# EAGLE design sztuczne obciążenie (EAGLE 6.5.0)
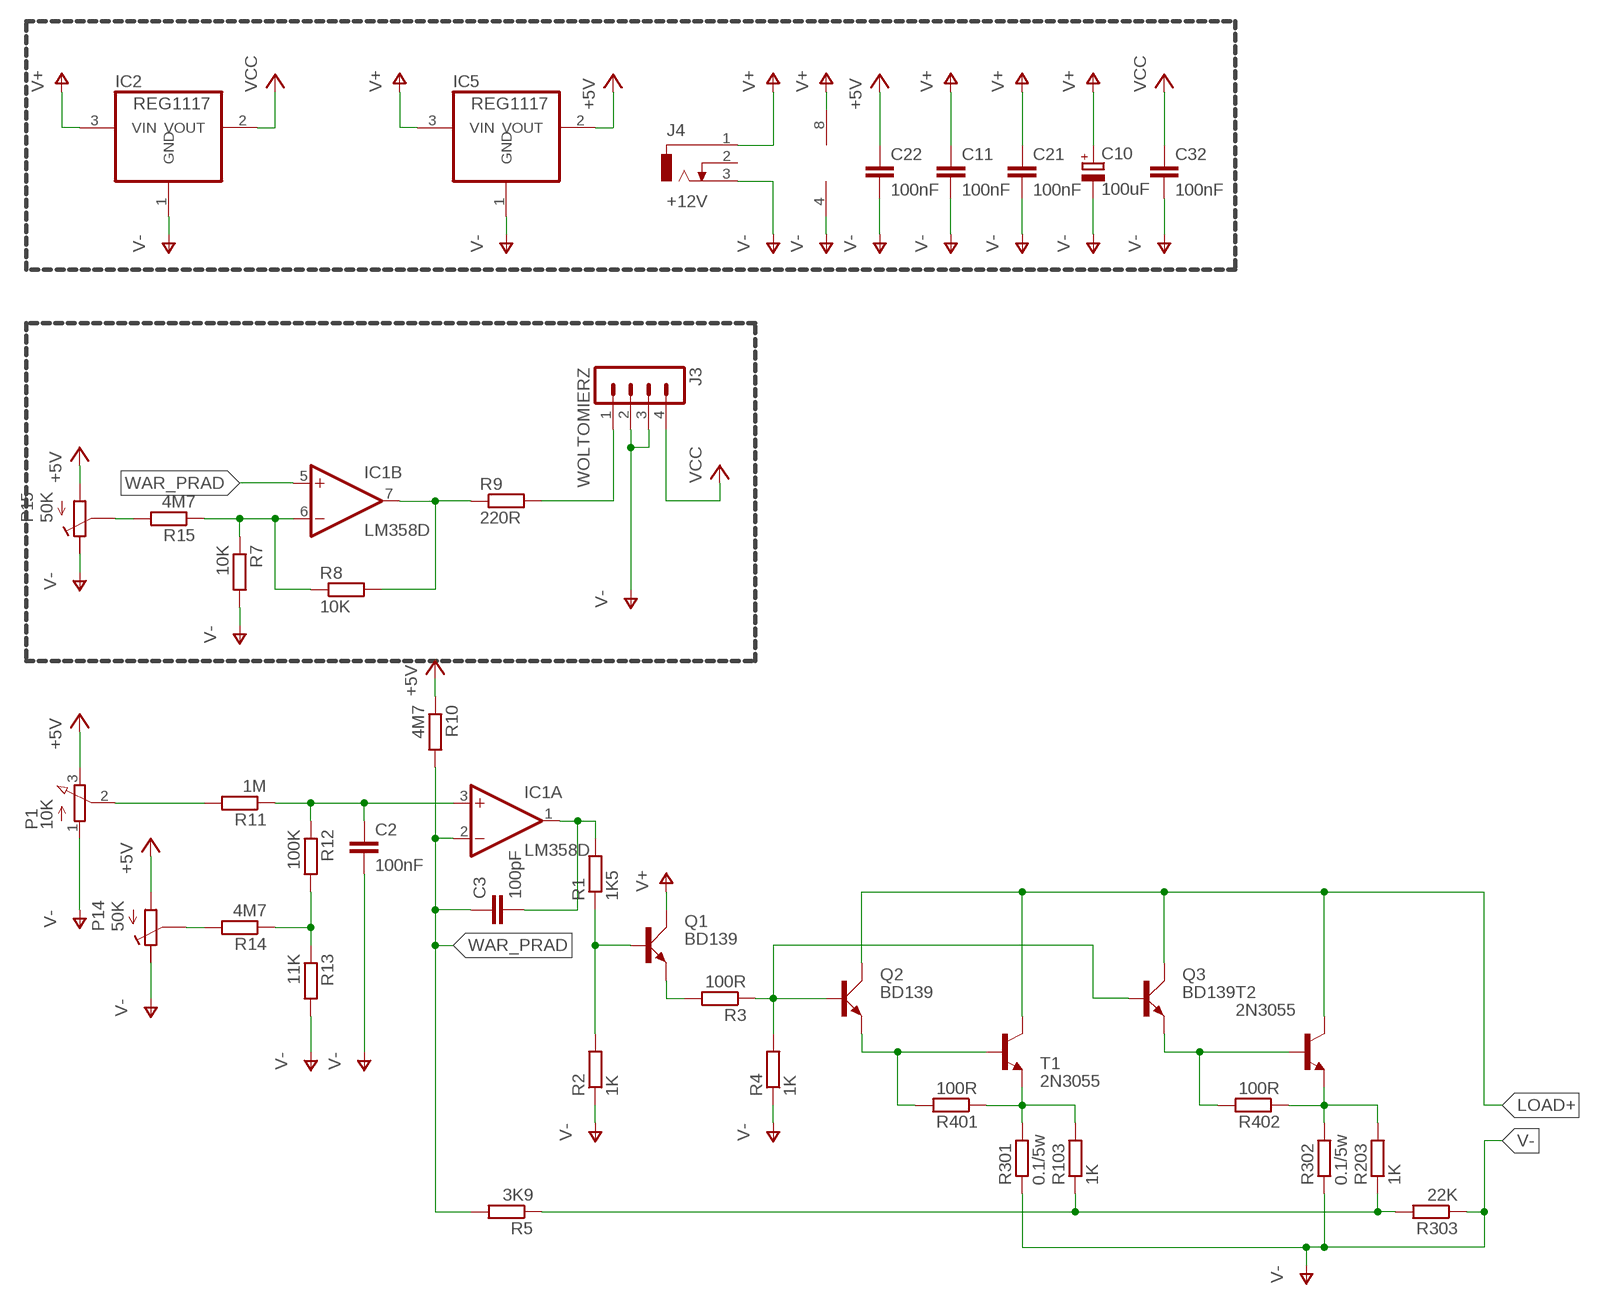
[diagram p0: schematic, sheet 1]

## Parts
C2  100nF  C-EU050-025X075  [C050-025X075]
C3  100pF  C-EUC1206K  [C1206K]
C10  100uF  CPOL-EUE5-10.5  [E5-10,5]
C11  100nF  C-EU050-025X075  [C050-025X075]
C21  100nF  C-EU050-025X075  [C050-025X075]
C22  100nF  C-EU050-025X075  [C050-025X075]
C32  100nF  C-EU050-025X075  [C050-025X075]
IC1  LM358D  [SO08]
IC2  REG1117  [SOT223]
IC5  REG1117  [SOT223]
J3  WOLTOMIERZ  MA04-1  [MA04-1]
J4  +12V  DCJ0202  [DCJ0202]
P1  10K  3RP/1610N  [3RP/1610N]
P14  50K  POTENCJOMETR_RM-065  [RM065]
P15  50K  POTENCJOMETR_RM-065  [RM065]
Q1  BD139  [TO126AV]
Q2  BD139  [TO126AV]
Q3  BD139  [TO126AV]
R1  1K5  R-EU_0207/7  [0207/7]
R2  1K  R-EU_0207/7  [0207/7]
R3  100R  R-EU_0207/7  [0207/7]
R4  1K  R-EU_0207/7  [0207/7]
R5  3K9  R-EU_0207/7  [0207/7]
R7  10K  R-EU_0207/7  [0207/7]
R8  10K  R-EU_0207/7  [0207/7]
R9  220R  R-EU_0207/7  [0207/7]
R10  4M7  R-EU_0207/7  [0207/7]
R11  1M  R-EU_0207/7  [0207/7]
R12  100K  R-EU_0207/7  [0207/7]
R13  11K  R-EU_0207/7  [0207/7]
R14  4M7  R-EU_0207/7  [0207/7]
R15  4M7  R-EU_0207/7  [0207/7]
R103  1K  R-EU_0207/7  [0207/7]
R203  1K  R-EU_0207/7  [0207/7]
R301  0.1/5w  R-EU_0922/22  [0922/22]
R302  0.1/5w  R-EU_0922/22  [0922/22]
R303  22K  R-EU_0207/7  [0207/7]
R401  100R  R-EU_0207/7  [0207/7]
R402  100R  R-EU_0207/7  [0207/7]
T1  2N3055  [TO3]
T2  2N3055  [TO3]

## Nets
+5V: C22.1 IC5.2(VOUT) P1.3(E) P14.P$3(A) P15.P$3(A) R10.1
LOAD+: Q2.C Q3.C T1.C T1.C/(C) T2.C T2.C/(C)
N$1: R103.2 R301.2 R401.1 T1.E
N$2: R203.2 R302.2 R402.1 T2.E
N$3: Q2.B Q3.B R3.1 R4.2
N$4: Q2.E R401.2 T1.B
N$5: Q1.B R1.1 R2.2
N$7: J3.1 R9.2
N$8: C3.2 IC1.1(A:OUT) R1.2
N$9: P1.2(S) R11.2
N$10: C2.1 IC1.3(A:+IN) R11.1 R12.1
N$11: R12.2 R13.1 R14.1
N$12: Q1.E R3.2
N$13: Q3.E R402.2 T2.B
N$14: R5.1 R103.1 R203.1 R303.2
N$15: P14.P$1(S) R14.2
N$16: IC1.6(B:-IN) R7.1 R8.1 R15.1
N$17: P15.P$1(S) R15.2
N$19: IC1.7(B:OUT) R8.2 R9.1
V+: C10.+ C11.1 C21.1 IC1.8(P:V+) IC2.3(VIN) IC5.3(VIN) J4.1 Q1.C
V-: C2.2 C10.- C11.2 C21.2 C22.2 C32.2 IC1.4(P:V-) IC2.1(GND) IC5.1(GND) J3.2 J3.3 J4.3 P1.1(A) P14.P$2(E) P15.P$2(E) R2.1 R4.1 R7.2 R13.2 R301.1 R302.1 R303.1
VCC: C32.1 IC2.2(VOUT) J3.4
WAR_PRAD: C3.1 IC1.2(A:-IN) IC1.5(B:+IN) R5.2 R10.2
Unconnected: J4.2

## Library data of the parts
C2 C3 C11 C21 C22 C32 = rcl:C-EU: CAPACITOR, European symbol
C10 = rcl:CPOL-EU: POLARIZED CAPACITOR, European symbol
IC1 = linear:LM358: OP AMP also LM158; LM258; LM2904 Source: http://cache.national.com/ds/LM/LM158.pdf
IC2 IC5 = burr-brown:REG1117: 800mA and 1A Low Dropout (LDO) Positive Regulator 1.8V, 2.5V, 2.85V, 3.3V, 5V, and Adj; MPN: REG1117; OC_FARNELL: 1097566; OC_NEWARK: 14P6981
J3 = con-lstb:MA04-1: PIN HEADER; OC_FARNELL: unknown; OC_NEWARK: unknown
J4 = con-jack:DCJ0202: DC POWER JACK Source: DCJ0202.pdf; OC_FARNELL: unknown; OC_NEWARK: unknown
P1 = pot:3RP/1610N: 16mm Potentiometer one level Source: http://www.alphapotentiometers.net/html/16mm_pot_2.html
P14 P15 = POT_RM065:POTENCJOMETR_RM-065
Q1-Q3 = transistor-power:BD139: NPN TRANSISTOR
R1-R5 R7-R15 R103 R203 R301-R303 R401 R402 = resistor:R-EU_: RESISTOR, European symbol
T1 T2 = transistor:2N3055: NPN TRANSISTOR

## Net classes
1 pradowa: width 1.524 mm, clearance 0.508 mm
2 srednia: width 0.635 mm

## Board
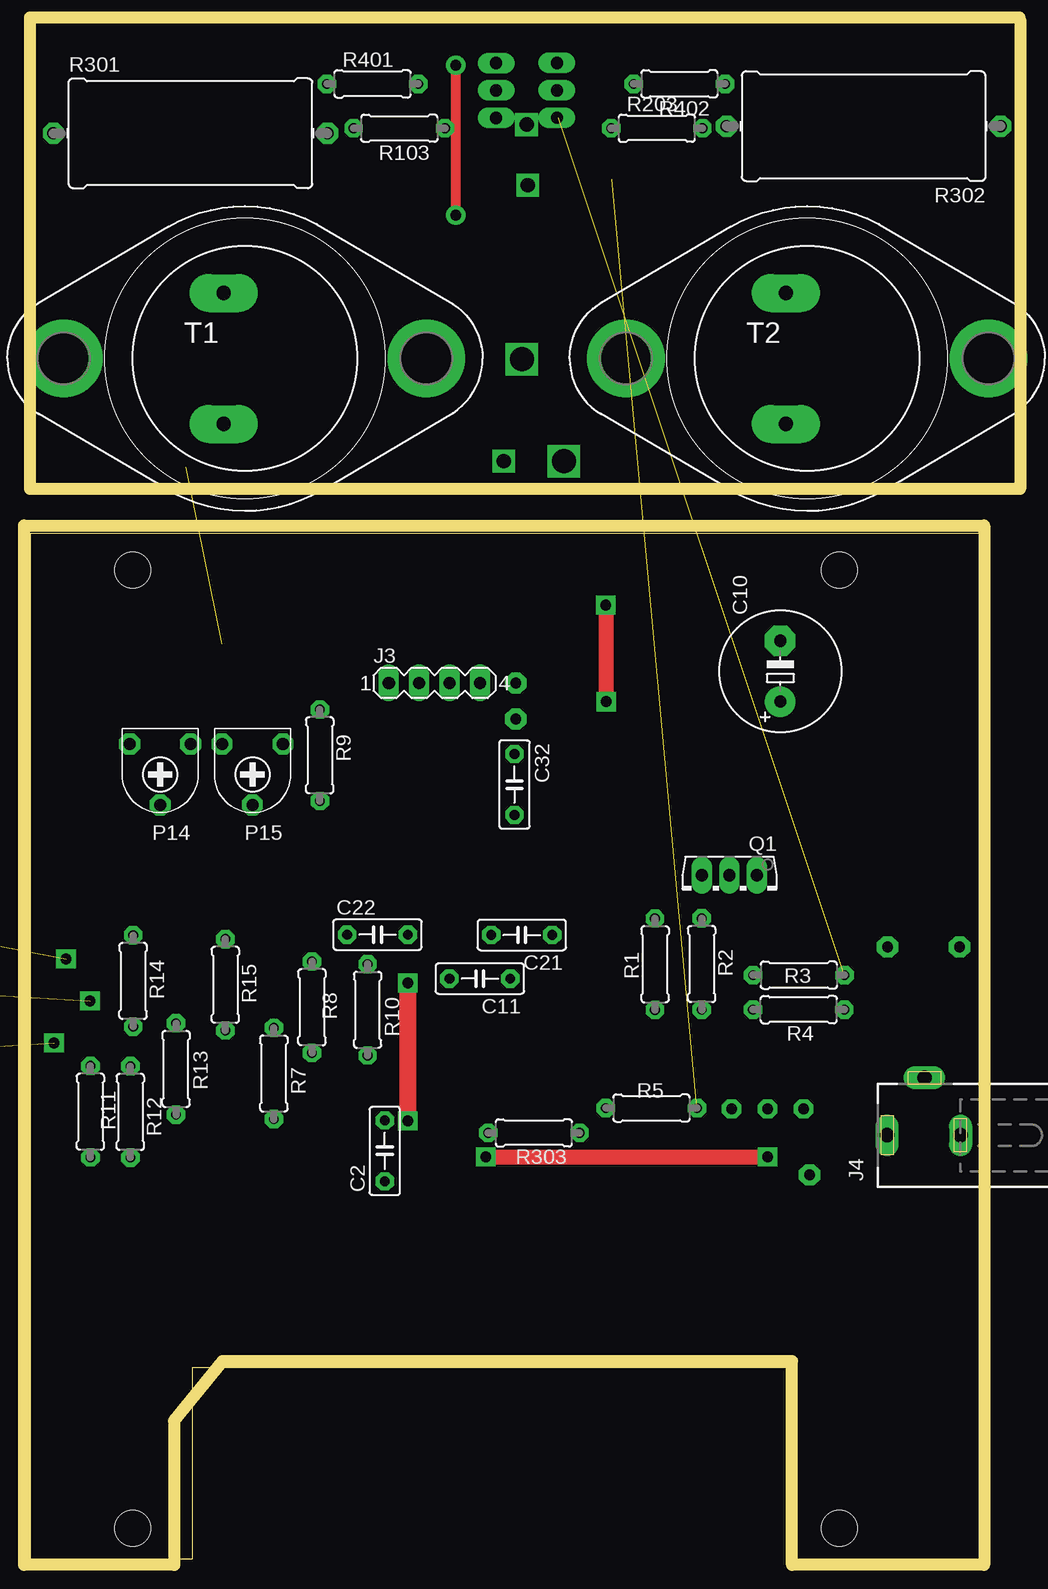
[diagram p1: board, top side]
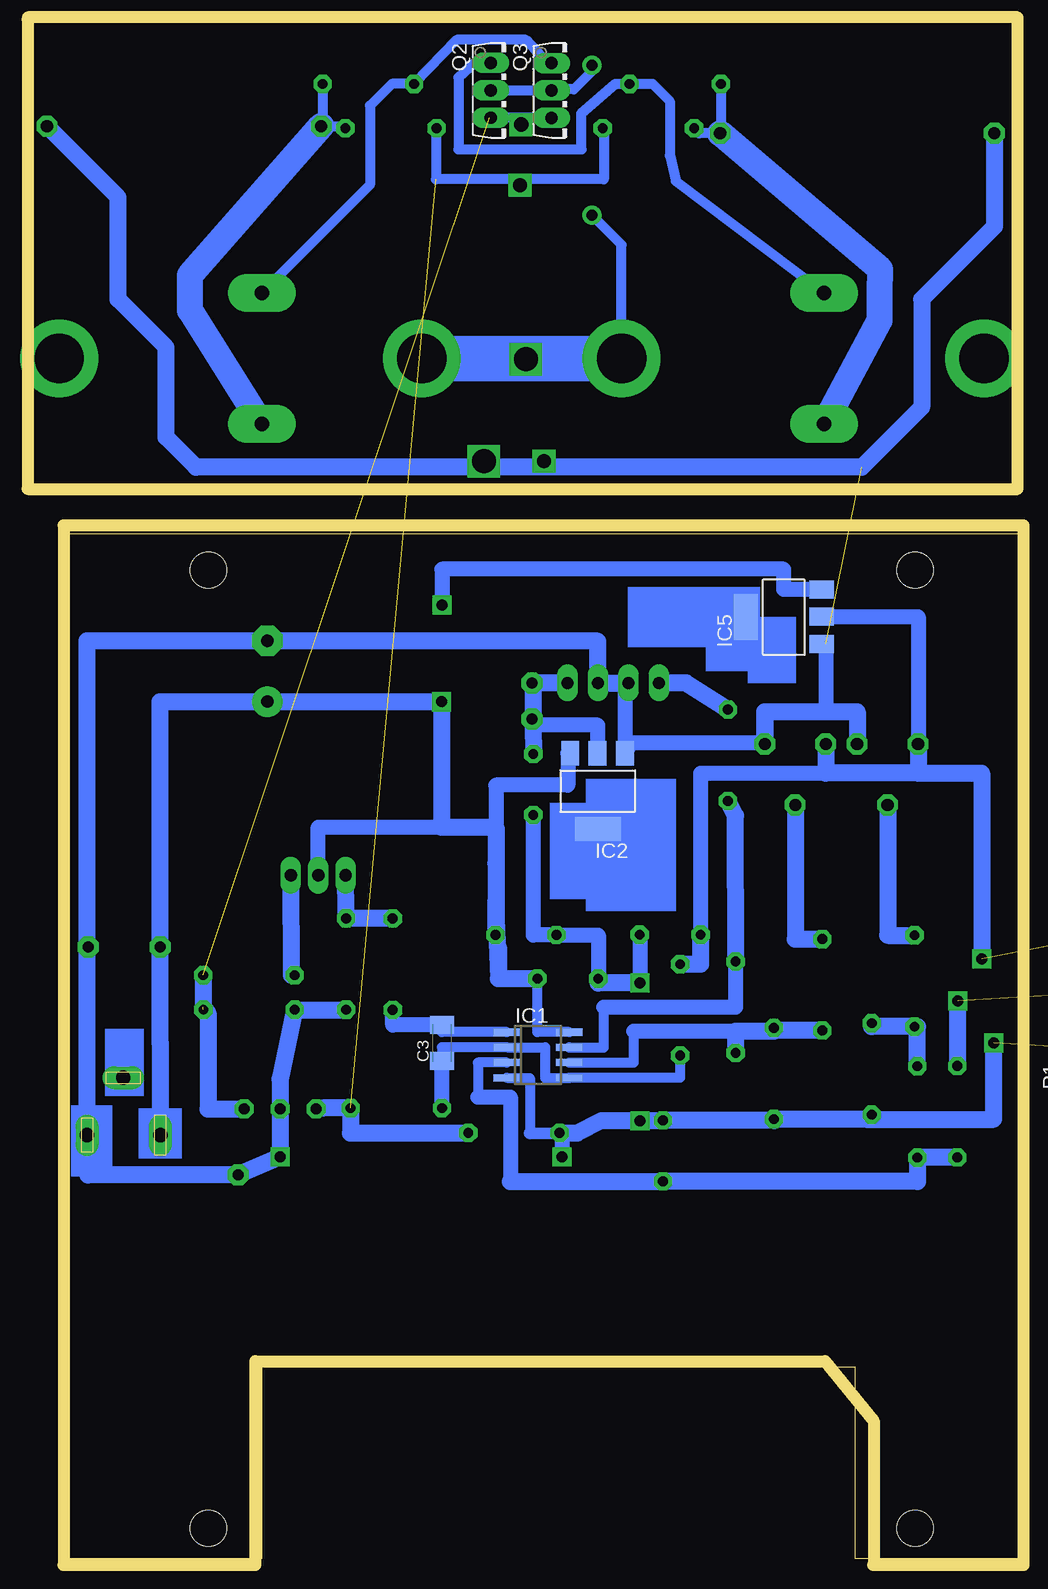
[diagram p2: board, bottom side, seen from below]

Size 79.22 x 85.48 mm. Coordinates in mm from the lower left corner, seen from the top.
Outline: 0,0 13.55,0 13.55,15.97 63.04,15.97 63.04,0 79.22,0 79.22,85.48 0,85.48 0,0
Copper layers (1*16): Top 0.035mm / dielectric 1.5mm / Bottom 0.035mm
Design rules "moj3_jeszcze_wieksze": minimum track width 23mil, minimum drill 23mil, track to track 16mil, track to pad 16mil, pad to pad 16mil, via to via 16mil, smd to smd 16mil, copper to edge 20mil, drill to drill 20mil, minimum pad ring 14mil, minimum via ring 14mil, stop-mask expansion 6mil, vias tented up to drill 0mil, thermal gap 13mil
Holes 3 mm at 8.56,2.54 67.48,2.54 67.48,82.42 8.56,82.42
Milling: 14 lines

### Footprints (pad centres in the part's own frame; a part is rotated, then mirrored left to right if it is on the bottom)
C050-025X075 = drill 0.813 octagon: 1 -2.54,0; 2 2.54,0
C1206K = smd 1.5 x 2: 1 -1.5,0; 2 1.5,0
E5-10,5 = drill 1.016 pad 2.54: + -2.54,0 | drill 1.016 pad 2.54 octagon: - 2.54,0
SO08 = smd 0.6 x 2.2: 1 -1.905,-2.6; 2 -0.635,-2.6; 3 0.635,-2.6; 4 1.905,-2.6; 5 1.905,2.6; 6 0.635,2.6; 7 -0.635,2.6; 8 -1.905,2.6
SOT223 = smd 1.499 x 2.007: 1 -2.261,-3.15; 2 0.025,-3.15; 3 2.311,-3.15 | smd 3.81 x 2.007: 4 0,3.15
MA04-1 = drill 1.016 long: 1 -3.81,0; 2 -1.27,0; 3 1.27,0; 4 3.81,0
DCJ0202 = drill 1.2 pad 1.93 long: 1 0,3.105; 2 4.8,0; 3 0,-3.015
3RP/1610N = drill 1.2 pad 2.184: 1 -5,0; 2 0,0; 3 5,0
RM065 = drill 1.016 octagon: P$1 0,2.54; P$2 -2.54,-2.54; P$3 2.54,-2.54
TO126AV = drill 1.016 long: B 2.286,-1.27; C 0,-1.27; E -2.286,-1.27
0207/7 = drill 0.813 octagon: 1 -3.81,0; 2 3.81,0
0922/22 = drill 1.016 octagon: 1 -11.43,0; 2 11.43,0
TO3 = drill 1.194 pad 3.15 long: B -1.778,5.461; E -1.778,-5.461 | drill 4.115 pad 6.477: C 15.113,0; C/ -15.113,0

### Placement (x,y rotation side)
C2  29.58,34 90 top
C3  48,43 90 bottom
C10  62.56,73.99 90 top
C11  37.51,48.36 180 top
C21  41,52 180 top
C22  28.97,52.03 0 top
C32  40.39,64.55 270 top
IC1  40,42 270 bottom
IC2  35,64 180 bottom
IC5  19.5,78.5 90 bottom
J3  33.72,73.01 0 top
J4  74.58,35.3 90 top
P1  not placed on the board
P14  10.85,65.38 180 top
P15  18.55,65.38 180 top
Q1  58.32,55.72 180 top
Q2  42.66,122.4 270 bottom  (outside the outline)
Q3  37.59,122.4 270 bottom  (outside the outline)
R1  52.11,49.56 270 top
R2  56,49.58 90 top
R3  64.1,48.65 180 top
R4  64.09,45.78 0 top
R5  51.81,37.57 180 top
R7  20.33,40.45 270 top
R8  23.51,45.98 90 top
R9  24.16,66.98 90 top
R10  28.15,45.76 270 top
R11  5.04,37.27 90 top
R12  8.37,37.25 90 top
R13  12.17,40.83 270 top
R14  8.6,48.17 90 top
R15  16.29,47.85 90 top
R103  30.79,119.25 180 top  (outside the outline)
R203  52.26,119.25 0 top  (outside the outline)
R301  13.38,118.83 0 top  (outside the outline)
R302  69.5,119.42 180 top  (outside the outline)
R303  42.01,35.5 0 top
R401  28.56,122.95 0 top  (outside the outline)
R402  54.14,122.95 180 top  (outside the outline)
T1  17.92,100.06 0 top  (outside the outline)
T2  64.8,100.06 0 top  (outside the outline)

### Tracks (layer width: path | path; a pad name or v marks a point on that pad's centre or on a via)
+5V  (via drill 0.9 pad 1.27)  (1 unrouted)
  Bottom 1.27: C22.1 26.43,65.5 16.01,65.5 | IC5.2 8.31,78.53 P14.P$3
  Bottom 1.422: P15.P$3 16.01,65.5 8.31,65.5 | P14.P$3 8.31,65.5 | R10.1 26.43,49.57 C22.1 | 8.31,65.5 3,65.5 v3,50
LOAD+  (via drill 0.9 pad 1.02)
  Top 0.813: v35.5,112 v35.5,124.5
  Bottom 0.813: Q2.C 38.48,122.4 Q3.C 38.76,122.5 37,122.5 35.5,124 v35.5,124.5 | T1.C 33.03,109.53 v35.5,112
  Bottom 3.81: T1.C T2.C/
N$1
  Bottom 0.813: R103.2 26.57,118.83 R301.2 24.75,118.89 R401.1
  Bottom 2.184: T1.E 11.5,103.24 11.5,105.5 11.47,107.5 R301.2
N$2
  Bottom 0.813: R203.2 56.24,119.42 R302.2 57.95,119.54 R402.1
  Bottom 2.184: T2.E 69,104.08 69,106.99 R302.2
N$3  (via drill 0.9 pad 1.42)  (2 unrouted)
  Bottom 0.813: Q3.B 44.05,120.11 Q2.B
  Bottom 1.422: R3.1 67.91,46 67.5,45.5 67.5,37.5 v64.5,37.5
N$4
  Bottom 0.813: T1.B 28.51,114.84 29,117 29,121.5 30.45,122.95 R401.2 33.55,122.95 36.38,120.5 36.38,118 36.37,117.5 46.63,117.5 46.63,123.5 45.31,124.69 Q2.E
N$5
  Bottom 1.422: R1.1 52.11,53.39 R2.2 56,53.81 Q1.B
N$6  (via drill 0.9 pad 1.78)
  other vias: 77.5,51
N$7
  Bottom 1.422: R9.2 27.66,73.01 J3.1
N$8
  Bottom 0.813: IC1.1 48,43.91 C3.2
  Bottom 1.27: C3.2 52.11,44.5 R1.2
N$9  (via drill 0.9 pad 1.27)  (1 unrouted)
  Bottom 1.422: R11.2 5,41.08 v5,46.5
N$10
  Bottom 0.813: IC1.3 45,41.37 45,38.5
  Bottom 1.27: 45,38.5 42.31,38.5 42.31,31.46
  Bottom 1.422: 42.31,31.46 C2.1 8.37,31.46 R12.1 5.04,33.44 R11.1
N$11
  Bottom 1.422: R13.1 12.17,44.36 R14.1 8.37,44.36 R12.2
N$12
  Bottom 1.422: Q1.E 60.58,48.65 R3.2
N$13
  Bottom 0.813: T2.B 54,114.54 54,121.14 52.19,122.95 R402.2 46.78,126.63 41,126.63 39.19,124.69 Q3.E
N$14  (via drill 0.9 pad 1.42)  (1 unrouted)
  Bottom 0.813: R103.1 34.5,119.15 34.5,115 48.5,115 48.45,115.05 R203.1
  Bottom 1.422: R303.2 55.62,35.5 R5.1 57.93,37.57 v58.5,37.5
N$15
  Bottom 1.422: P14.P$1 10.85,51.98 R14.2
N$16
  Bottom 0.813: IC1.6 32,41.37 32,44
  Bottom 1.27: 32,44 23.5,44
  Bottom 1.422: R15.1 20.33,44.04 | 20.33,44.04 R7.1 | R8.1 23.5,43.67 23.5,44 20.33,44 20.33,44.04
N$17
  Bottom 1.422: P15.P$1 18.55,51.66 R15.2
N$18  (via drill 0.9 pad 1.78)
  other vias: 40.5,73
N$19
  Bottom 0.813: IC1.7 34.5,42.62 34.5,46
  Bottom 1.27: 34.5,46 23.5,46 23.5,47 23.51,47 R8.2
  Bottom 1.422: R8.2 23.53,61.94 R9.1
N$20  (via drill 2)
  other vias: 41,100
N$21  (via drill 1.2)
  other vias: 39.5,91.5
N$22  (via drill 1.2)
  other vias: 41.5,114.5
N$23  (via drill 1.2)
  other vias: 41.4,119.55
N$24  (via drill 2)
  other vias: 44.5,91.5
N$25  (via drill 0.9 pad 1.78)
  other vias: 40.5,70
V+  (via drill 0.9, 0.9 pad 1.78)
  Top 1.27: v48,79.5 48.04,79.5 v48.04,71.45
  Bottom 0.813: IC1.8 40.05,43.91 C11.1
  Bottom 1.27: IC2.3 37.5,67.15 37.5,64.5 43.5,64.5 43.5,61 | IC5.3 19.5,80.81 19.5,82.5 48,82.5 v48,79.5 | Q1.C 58.32,61 48.04,61
  Bottom 1.422: J4.1 71.47,43 71.5,43 v71.5,51 71.5,71.45 C10.+ v48.04,71.45 48.04,61 43.5,61 43.5,58 | 43.5,58 C21.1 | 43.5,58 43.5,53.36 43.31,48.36 | 43.31,48.36 C11.1 | 43.31,51 43.31,48.36
V-  (via drill 0.9, 0.9 pad 1.27, 0.9 pad 1.42, 0.9 pad 1.78)  (2 unrouted)
  Top 1.27: v38,33.5 v61.5,33.5
  Top 1.422: v31.5,36.5 v31.5,48
  Bottom 0.813: IC1.4 40.68,40.07 40.68,35.48 | v31.5,36.5 29.58,36.5 C2.2
  Bottom 1.016: 40.68,35.48 R303.1
  Bottom 1.27: 38,35.5 v38,33.5 | J3.2 32.74,73.01 32.74,67.5 | 32.74,67.5 IC2.1 | C32.2 40.39,52 C21.2 34.97,52 C11.2 | 21.09,70.61 21,70.61 21,68 32.5,68 32.5,67.5 32.74,67.5 | IC5.1 16,76.24 16,70.61 | C22.2 v31.5,48
  Bottom 1.422: R4.1 60.28,45.77 R2.1 | 60.3,45.78 R4.1 | 21.09,68.5 P15.P$2 21.09,70.61 16,70.61 13.39,70.61 P14.P$2 | 32.5,73.01 J3.2 J3.3 35,76.5 62.56,76.5 C10.- 77.59,76.53 J4.3 77.5,35.8 77.5,32 v65,32 v61.5,33.5 v61.5,37.5 61.5,40 R4.1 | R13.2 12.67,36.64 | 12.67,36.64 R7.2 20.33,36.54 C2.2 34.69,36.54 36.73,35.5 38,35.5 R303.1 | v31.5,48 34.97,48 C11.2 | 12.67,36.64 2,36.64 v2,43 | R301.1 1.95,111.05 8,105 8,96 13,91 68.5,91 71,93.5 71,101 75,105 75,113.49 R302.1
VCC
  Bottom 1.27: IC2.2 35,67.15 35,69.5 40.4,69.5
  Bottom 1.422: 40.41,73.01 40.4,69.5 C32.1 | J3.4 40.41,73.01 | 40.41,73.01 40.41,73.04
WAR_PRAD
  Bottom 0.813: C3.1 48,42.63 IC1.2 39.4,42.63 39.4,40.08 IC1.5 28.15,40.09 R10.2
  Bottom 1.27: R5.2 C3.1
  Bottom 1.422: R5.2
(copper drawn outside any net)
  shapes: Bottom area x8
